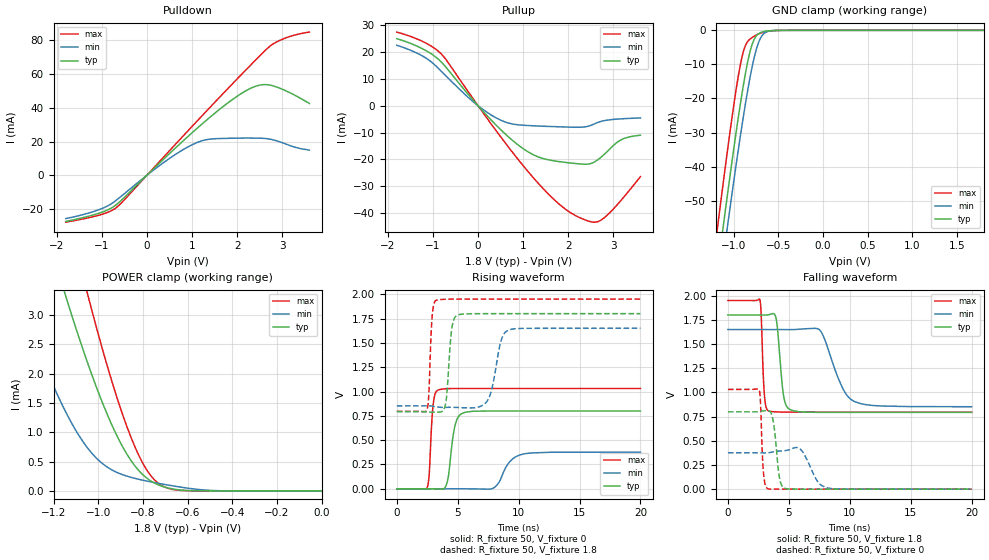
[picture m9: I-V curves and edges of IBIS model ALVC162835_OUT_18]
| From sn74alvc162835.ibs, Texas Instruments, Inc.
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[Model]   ALVC162835_OUT_18
Model_type  3-state
Enable   Active-Low
Vref =   0
Rref =   1000
Cref =   30p
Vmeas =   0.9
| variable   typ   min   max
C_comp   6.23pF   5.25pF   7.43pF
| C_pullup   5.60pF   3.87pF   7.72pF
| C_pulldown   4.82pF   3.49pF   7.13pF
| C_tri-state   6.23pF   5.25pF   7.43pF
[Temperature Range]   40   100   -40
| Ambient temperature   25   85   -40
[Voltage range]   1.8   1.65   1.95
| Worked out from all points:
|   slope of the pulldown table from 0 to 0.27 V, typ, clamps not added: 38.6 ohm
|   slope of the pullup table from 0 to 0.27 V, typ, clamps not added: 54.5 ohm
|   GND clamp passes 1 mA (typ) near -0.72 V on its own axis
|   POWER clamp passes 1 mA (typ) near -0.92 V on its own axis
|   rising waveform, R_fixture 50, V_fixture 0: 20-80 % time 490ps typ, 1.03ns min, 266ps max; typ from 0 V to 0.8 V
|   falling waveform, R_fixture 50, V_fixture 1.8: 20-80 % time 423ps typ, 1.45ns min, 208ps max; typ from 1.8 V to 0.793 V
|   rising waveform, R_fixture 50, V_fixture 1.8: 20-80 % time 345ps typ, 721ps min, 223ps max; typ from 0.793 V to 1.8 V
|   falling waveform, R_fixture 50, V_fixture 0: 20-80 % time 387ps typ, 881ps min, 199ps max; typ from 0.8 V to 0 V
[GND Clamp]
| ALVC162835_OUT_18
|   Voltage   I(typ)   I(min)   I(max)
-1.8V     -201.4mA   -207.6mA   -191.8mA
-1.19V    -72.47mA   -81.34mA   -59.95mA
-1.17V    -68.41mA   -77.37mA   -55.8mA
-1.11V    -56.38mA   -65.58mA   -43.56mA
-1.065V   -47.53mA   -56.9mA    -34.62mA
-975mV    -30.53mA   -40.07mA   -17.95mA
-915mV    -20.06mA   -29.44mA   -8.904mA
-860mV    -11.61mA   -20.39mA   -4.057mA
-775mV    -2.963mA   -8.638mA   -1.806mA
-695mV    -630.7uA   -2.132mA   -797.9uA
-585mV    -87.28uA   -155.2uA   -156.9uA
1.8V      1.171nA    278.4pA    11.33nA
[POWER Clamp]
| ALVC162835_OUT_18
|   Voltage   I(typ)   I(min)   I(max)
-1.8V     13.29mA    8.861mA    17.2mA
-1.355V   6.151mA    3.289mA    8.476mA
-1.245V   4.612mA    2.188mA    6.529mA
-1.14V    3.259mA    1.307mA    4.783mA
-1.05V    2.213mA    744.4uA    3.395mA
-1.04V    2.104mA    695.6uA    3.248mA
-950mV    1.221mA    383.5uA    2.012mA
-860mV    558uA      239.4uA    981.4uA
-795mV    258.9uA    178.5uA    437.1uA
-735mV    110.6uA    132.9uA    143.8uA
-630mV    14.79uA    64.43uA    8.958uA
-16.28fV  1.171nA    35.77pA    11.21nA
[Pulldown]
| ALVC162835_OUT_18
|   Voltage   I(typ)   I(min)   I(max)
-1.8V     -27.42mA   -25.72mA   -27.83mA
-1.05V    -22.39mA   -20.29mA   -23.59mA
-650mV    -16.81mA   -14.19mA   -18.54mA
365mV     9.416mA    7.421mA    10.63mA
1.04V     26.11mA    18.57mA    30.07mA
1.415V    34.8mA     21.46mA    40.73mA
1.915V    45.26mA    21.95mA    54.74mA
2.29V     51.43mA    22.04mA    65.06mA
2.575V    53.72mA    21.89mA    72.76mA
2.845V    52.57mA    20.63mA    78.6mA
3.19V     48.64mA    17.42mA    82.44mA
3.6V      42.56mA    14.91mA    84.87mA
[Pullup]
| ALVC162835_OUT_18
|   Voltage   I(typ)   I(min)   I(max)
-1.8V     24.92mA    22.48mA    27.38mA
-1.205V   20.96mA    18.24mA    23.71mA
-815mV    16.26mA    12.81mA    19.25mA
-65mV     1.244mA    880.5uA    1.546mA
490mV     -8.71mA    -5.288mA   -11.32mA
1.255V    -18.5mA    -7.509mA   -27.37mA
1.715V    -20.6mA    -7.809mA   -35.38mA
2.1V      -21.41mA   -8.008mA   -40.32mA
2.465V    -21.67mA   -7.525mA   -43.02mA
2.705V    -19.46mA   -5.956mA   -42.78mA
3.15V     -12.89mA   -4.918mA   -35.6mA
3.6V      -10.98mA   -4.555mA   -26.38mA
[Ramp]
| ALVC162835_OUT_18
| variable   typ   min   max
dV/dt_r   0.48/4.93E-10   0.23/1.03E-09   0.62/2.80E-10
dV/dt_f   0.61/4.34E-10   0.49/1.46E-09   0.70/2.19E-10
R_load = 50
[Rising Waveform]
| ALVC162835_OUT_18
R_fixture =   50
C_fixture =   0
L_fixture =   0
V_fixture =   0
V_fixture_min = 0
V_fixture_max = 0
|   Time   V(typ)   V(min)   V(max)
0s        12.63pV    43.22pV    9.526pV
2.505ns   217.4uV    -2.601uV   17.7mV
2.985ns   -83.22uV   650.8uV    865mV
3.425ns   -1.397mV   270.8uV    1.017V
4.1ns     53.16mV    -98.72uV   1.029V
4.77ns    645.4mV    132.8uV    1.031V
5.44ns    779.5mV    229uV      1.031V
7.935ns   799.4mV    7.853mV    1.031V
10.4ns    799.5mV    358mV      1.031V
20ns      799.5mV    376.1mV    1.031V
[Falling Waveform]
| ALVC162835_OUT_18
R_fixture =   50
C_fixture =   0
L_fixture =   0
V_fixture =   1.8
V_fixture_min = 1.65
V_fixture_max = 1.95
|   Time   V(typ)   V(min)   V(max)
0s        1.8V       1.65V      1.95V
2.615ns   1.799V     1.65V      1.96V
2.99ns    1.8V       1.65V      981.2mV
3.355ns   1.803V     1.649V     806.3mV
3.955ns   1.766V     1.65V      798.7mV
4.56ns    973.8mV    1.65V      796.8mV
5.12ns    821.5mV    1.649V     796.3mV
7.545ns   793.9mV    1.644V     796.1mV
10.47ns   793.2mV    901.3mV    796.1mV
20ns      793.2mV    852mV      796.1mV
[Rising Waveform]
| ALVC162835_OUT_18
R_fixture =   50
C_fixture =   0
L_fixture =   0
V_fixture =   1.8
V_fixture_min = 1.65
V_fixture_max = 1.95
|   Time   V(typ)   V(min)   V(max)
0s        793.2mV    852mV      796.1mV
2.48ns    787.8mV    853.3mV    816.4mV
2.905ns   787.2mV    849.3mV    1.776V
3.24ns    787.1mV    842.2mV    1.938V
3.98ns    857.6mV    837mV      1.948V
4.5ns     1.634V     837.6mV    1.95V
4.98ns    1.785V     836.1mV    1.95V
7.445ns   1.8V       906.7mV    1.95V
9.17ns    1.8V       1.63V      1.95V
20ns      1.8V       1.65V      1.95V
[Falling Waveform]
| ALVC162835_OUT_18
R_fixture =   50
C_fixture =   0
L_fixture =   0
V_fixture =   0
V_fixture_min = 0
V_fixture_max = 0
|   Time   V(typ)   V(min)   V(max)
0s        799.5mV    376.1mV    1.031V
2.57ns    801.1mV    375.5mV    1.024V
2.925ns   809.4mV    374.6mV    161.6mV
3.295ns   812.4mV    376mV      4.191mV
3.675ns   730.5mV    384.6mV    1.015mV
4.215ns   131.9mV    393.7mV    340.9uV
4.64ns    10.21mV    397.5mV    119.1uV
5.935ns   313.8uV    414mV      6.182uV
8.23ns    10.95uV    11.26mV    61.38nV
20ns      -3.662nV   595.2nV    -1.257nV
